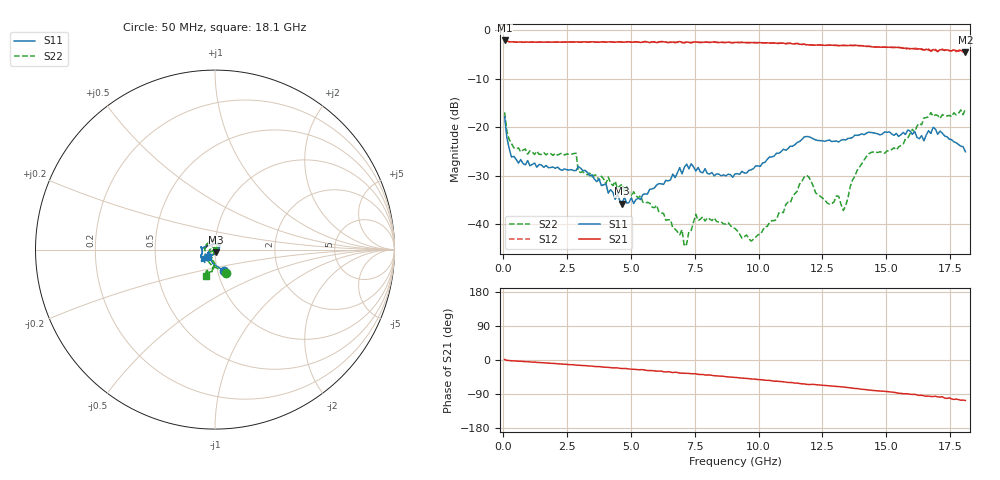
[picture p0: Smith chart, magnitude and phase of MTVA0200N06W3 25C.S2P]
! Network Analyzer HP8720D.06.14 Serial No. US36140669
! 19 Aug 2005  14:19:07
! Frequency  S11  S21  S12  S22
# HZ  S  DB R 50
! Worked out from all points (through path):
!   201 points, 50 MHz to 18.1 GHz, reference 50 ohm
!   highest |S21| = -2.10 dB at 50 MHz (marker M1); lowest = -4.5 dB at 18.1 GHz (marker M2)
!   group delay of S21, straight-line fit = 16.2 ps
!   lowest |S11| = -35.8 dB at 4.653 GHz (marker M3), VSWR 1.03, Z = 50.6 - j1.5 ohm
!   |S11| at or under -10 dB: start of sweep to end of sweep
!   |S22| runs from -44.6 to -16.2 dB; largest |S21 - S12| = 0.027
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5e7  -17.81 -67.5  -2.10 1.4  -2.13 1.5  -16.94 -64.9
3.2075e8  -26.18 -127.3  -2.40 -2.2  -2.39 -2.1  -23.40 -138.4
5.915e8  -27.43 -147.2  -2.43 -3.3  -2.43 -3.1  -24.28 -166.9
2.84775e9  -28.98 -149.4  -2.40 -13.6  -2.43 -13.3  -25.37 89.4
2.938e9  -28.12 -130.5  -2.41 -13.8  -2.42 -14.1  -29.14 89.2
3.1185e9  -28.99 -126.7  -2.40 -14.7  -2.46 -14.6  -29.23 83.9
4.65275e9  -35.83 -66.1  -2.45 -22.5  -2.42 -22.4  -31.80 54.4
6.09675e9  -31.66 19.8  -2.45 -29.2  -2.37 -29.3  -37.57 38.4
6.99925e9  -29.65 50.3  -2.49 -34.8  -2.57 -35.3  -41.17 55.7
7.0895e9  -28.29 45.7  -2.62 -35.0  -2.51 -34.9  -44.58 75.6
7.54075e9  -29.07 47.5  -2.40 -36.4  -2.35 -37.4  -38.00 111.0
9.075e9  -29.66 107.4  -2.50 -45.9  -2.50 -45.9  -40.90 136.8
9.70675e9  -28.80 135.6  -2.53 -50.1  -2.55 -49.6  -43.53 175.9
1.17825e10  -22.02 173.6  -2.87 -63.1  -2.88 -63.3  -30.34 -158.9
1.21435e10  -22.43 170.5  -3.07 -64.1  -3.05 -64.5  -32.21 177.2
1.313625e10  -23.07 -170.7  -3.19 -70.4  -3.13 -70.5  -34.27 -151.4
1.331675e10  -22.56 -165.4  -3.10 -71.2  -3.12 -71.6  -37.23 -138.5
1.421925e10  -21.25 -155.0  -3.33 -78.4  -3.32 -78.5  -26.12 -111.3
1.512175e10  -20.98 -149.8  -3.51 -84.0  -3.47 -84.0  -24.91 -111.1
1.64755e10  -22.82 -131.4  -4.09 -94.6  -4.06 -92.1  -18.10 -98.8
1.68365e10  -20.03 -140.1  -3.97 -96.4  -4.14 -98.0  -17.76 -105.3
1.81e10  -25.09 -134.1  -4.51 -106.8  -4.42 -107.6  -16.24 -109.3
